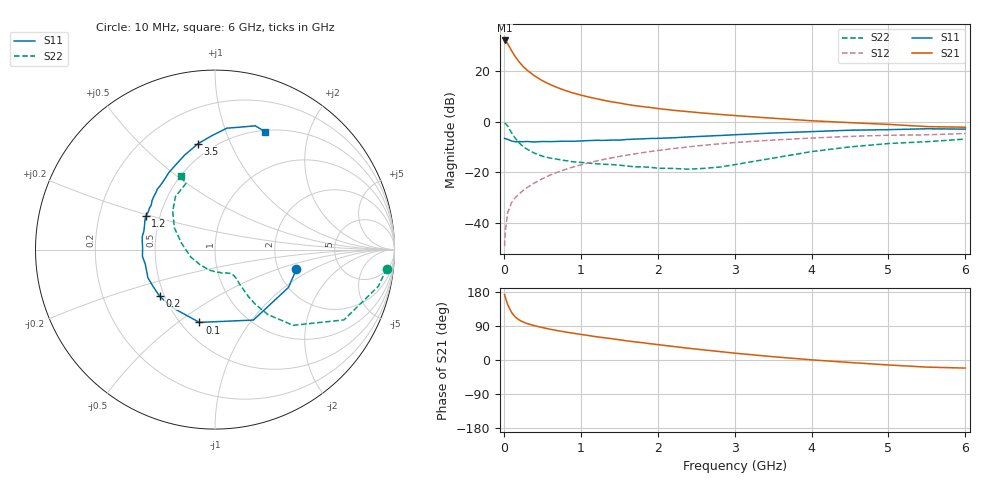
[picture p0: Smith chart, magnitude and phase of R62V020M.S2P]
! SIEMENS Small Signal Semiconductors
! BFR193
! Si NPN RF Bipolar Junction Transistor in SOT23
! VCE = 2 V  IC = 20 mA
! Common Emitter S-Parameters:  May  1996
# GHz  S  MA  R  50
!  f  S11  S21  S12  S22
! GHz  MAG  ANG  MAG  ANG  MAG  ANG  MAG  ANG
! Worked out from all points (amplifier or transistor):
!   36 points, 10 MHz to 6 GHz, reference 50 ohm
!   highest |S21| = 32.3 dB at 10 MHz (marker M1)
!   |S21| within 3 dB of that: start of sweep to 81.38 MHz
!   unconditionally stable (mu >= 1): 541.8 MHz to 1.854 GHz
!   at 250 MHz: K = 0.84, MSG = 24.6 dB, |S12| = -27.3 dB
!   at 1.4 GHz: K = 1.03, MAG = 10.1 dB, |S12| = -14.3 dB
!   at 6 GHz: K = 0.95, MSG = 1.2 dB, |S12| = -4.6 dB
!   lowest NFmin = 1.40 dB at 450 MHz
!   S11 on the Smith chart (normalised r, x): 10 MHz: 2.51, -0.71; 100 MHz: 0.62, -0.60; 200 MHz: 0.47, -0.29; 1.2 GHz: 0.42, +0.19; 3.5 GHz: 0.42, +0.76; 6 GHz: 0.52, +1.39
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0.01  0.4664 -13.7  41.01 172.5  0.0034 87.7  0.962 -6.3
0.02  0.4605 -27.2  40.28 164.8  0.0069 79.8  0.9332 -12.6
0.05  0.4471 -61.4  35.34 146.0  0.0157 70.6  0.8183 -28.6
0.1  0.4148 -102.1  25.84 125.4  0.0249 62.9  0.6062 -44.1
0.15  0.4002 -125.5  19.38 113.1  0.0314 62.0  0.4669 -50.8
0.2  0.4035 -139.9  15.32 105.6  0.0371 62.4  0.3797 -53.6
0.25  0.4015 -149.8  12.53 100.3  0.0432 64.1  0.3222 -54.6
0.3  0.4056 -157.2  10.62 96.3  0.0493 65.5  0.2865 -54.5
0.4  0.3968 -168.0  8.122 90.5  0.0613 67.5  0.2372 -54.6
0.5  0.406 -174.8  6.53 85.6  0.0739 68.4  0.2076 -53.7
0.6  0.4031 179.1  5.493 81.3  0.0873 68.7  0.1905 -53.6
0.7  0.4076 173.9  4.746 77.4  0.1001 68.4  0.1797 -53.9
0.8  0.4116 169.8  4.166 74.0  0.1131 67.9  0.1695 -55.0
0.9  0.4095 165.3  3.723 70.7  0.1265 67.4  0.1607 -55.9
1.1  0.4229 157.4  3.104 64.6  0.153 65.8  0.1515 -60.4
1.2  0.4282 154.2  2.873 61.5  0.1658 64.8  0.1468 -62.8
1.6  0.445 141.9  2.209 50.5  0.2178 60.0  0.1324 -76.2
2.2  0.4804 126.1  1.691 35.8  0.2936 51.9  0.1184 -106.4
3.5  0.5981 99.0  1.173 8.7  0.4333 31.9  0.1899 169.1
4.5  0.6798 84.4  0.96 -6.6  0.5123 17.6  0.3172 138.0
5.5  0.7251 72.0  0.802 -18.8  0.5499 3.2  0.4024 113.8
6  0.714 66.8  0.779 -21.3  0.5861 -1.0  0.4534 114.8
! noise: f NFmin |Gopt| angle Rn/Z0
0.45  1.4  0.3  160  0.1
0.9  1.45  0.34  172  0.11
1.8  2.2  0.56  -148  0.2
